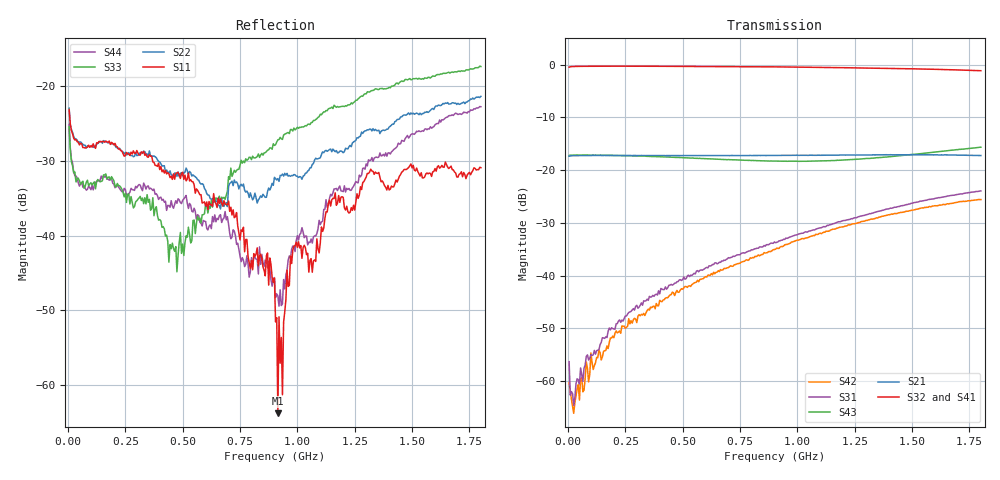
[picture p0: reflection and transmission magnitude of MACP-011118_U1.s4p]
!Agilent Technologies,E5071C,MY46110647,A.11.31
!Date: Thu Jan 18 12:34:23 2024 DD
!Data & Calibration Information:
!MACP-011118 soldered onto PT-0003645 with F connectors, Calibration PT-0003645-TRL. Port1 (pin3) Port2 (pin1) Port3 (pin6) Port4 (pin4)
!Freq	S11:SOLT4(ON)	S12:SOLT4(ON)	S13:SOLT4(ON)	S14:SOLT4(ON)
!	S21:SOLT4(ON)	S22:SOLT4(ON)	S23:SOLT4(ON)	S24:SOLT4(ON)
!	S31:SOLT4(ON)	S32:SOLT4(ON)	S33:SOLT4(ON)	S34:SOLT4(ON)
!	S41:SOLT4(ON)	S42:SOLT4(ON)	S43:SOLT4(ON)	S44:SOLT4(ON)
!PortZ  Port1:75+j0  Port2:75+j0  Port3:75+j0  Port4:75+j0
!Above PortZ is port z conversion or system Z0 setting when saving the data.
!When reading, reference impedance value at option line is always used.
# Hz S MA R 75
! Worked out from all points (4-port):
!   360 points, 5 MHz to 1.8 GHz, reference 75 ohm
!   strongest paths, dB at 5 MHz, 455 MHz, 905 MHz, 1.355 GHz, 1.8 GHz:
!     S32: -0.5, -0.3, -0.4, -0.7, -1.2
!     S41: -0.5, -0.3, -0.5, -0.7, -1.2
!     S21: -17.4, -17.3, -17.2, -17.1, -17.3
!     S43: -17.2, -17.6, -18.3, -17.6, -15.7
!     S31: -56.3, -41.8, -33.8, -27.8, -24.0
!     S42: -60.2, -43.1, -35.0, -28.9, -25.6
!   lowest |S11| = -63.8 dB at 915 MHz (marker M1), VSWR 1.00, Z = 74.9 + j0.069 ohm
!   |S11| at or under -10 dB: start of sweep to end of sweep
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5000000  0.06977 147.6  0.1342 -178.0  0.001266 -61.1  0.9464 2.2
         0.1353 -177.7  0.07129 148.8  0.9485 2.2  0.000391 -145.5
         0.001526 -86.2  0.9433 2.3  0.05348 133.2  0.1369 1.3
         0.9462 2.3  0.0009734 -59.7  0.1373 2.2  0.05541 136.4
3e7  0.04368 168.6  0.1368 178.6  0.0001664 128.9  0.9581 -0.1
     0.1369 178.6  0.04449 169.4  0.9583 -0.1  0.0006066 -173.0
     0.0006894 -179.3  0.9588 -0.2  0.02667 163.9  0.1385 -0.0
     0.9579 -0.1  0.0006234 -175.1  0.1385 0.1  0.0252 155.6
2.05e8  0.04147 170.6  0.1373 165.3  0.003878 102.5  0.9637 -5.6
        0.1375 165.3  0.04022 177.2  0.9643 -5.9  0.002743 114.9
        0.003097 115.0  0.964 -5.9  0.02161 -169.5  0.1373 -2.9
        0.9639 -5.6  0.002833 110.2  0.1374 -2.9  0.02094 158.2
8.7e8  0.007659 92.3  0.1375 118.3  0.01982 73.1  0.9499 -25.1
       0.1376 118.2  0.01973 -143.1  0.9499 -25.9  0.01607 84.3
       0.01963 79.7  0.9512 -25.9  0.03729 -91.6  0.1219 -5.1
       0.9495 -25.1  0.01651 81.8  0.1217 -5.0  0.006078 45.0
9.15e8  0.0006481 134.8  0.1377 115.2  0.02118 72.0  0.948 -26.4
        0.1376 115.1  0.02408 -138.8  0.9491 -27.3  0.0173 81.5
        0.02082 77.8  0.9501 -27.4  0.0438 -93.3  0.1213 -4.6
        0.9484 -26.4  0.01807 80.8  0.1215 -4.5  0.003965 24.0
1.165e9  0.01935 -30.0  0.1384 97.5  0.03098 60.9  0.9356 -33.7
         0.1383 97.6  0.03648 -113.7  0.9335 -35.1  0.02566 68.2
         0.03141 65.5  0.935 -35.2  0.07342 -92.8  0.1232 -0.6
         0.9357 -33.7  0.02759 66.3  0.1232 -0.7  0.02057 -59.3
1.8e9  0.02848 -126.4  0.1375 48.8  0.06287 20.7  0.8747 -53.4
       0.1372 48.8  0.08545 -145.3  0.8723 -55.3  0.04886 22.9
       0.06344 22.2  0.8741 -55.5  0.1354 -118.1  0.1642 -1.0
       0.8749 -53.4  0.05247 22.7  0.1645 -0.9  0.07285 -109.7
